[IBIS Ver]   5.0
[Comment Char] |_char
[File name]   dlpc231_ibis.ibs
[File Rev]   1.0
[Date]   August 11,2022
[Source]   Cadence SpeedXP Suite XtractIM 18.0.4.05011.160686   004
[Notes]   One-Section RLC
[Disclaimer]   The model given below represents a 201-pin package.
[Copyright]
[Component] Component_Name
[Manufacturer] Manufacturer_Name
[Package]
|   typ   min   max
R_pkg   0.29997   0.18892   0.43741
L_pkg   4.092e-9   2.338e-9   5.75e-9
C_pkg   1.277e-12   1.026e-12   1.843e-12
[Package Model]   dlpc231_pkg
[Pin]   Signal_name   model_name   R_pin   L_pin   C_pin
A1	GND18A_LVDS	GND
A10	DMD_LS0_CLK_N	fxslvtx-tx_n
A11	DMD_HS0_WDATA7_N	fxslvtx-tx_n
A12	DMD_HS0_WDATA6_N	fxslvtx-tx_n
A13	DMD_HS0_WDATA5_N	fxslvtx-tx_n
A14	DMD_HS0_WDATA4_N	fxslvtx-tx_n
A15	DMD_HS0_CLK_N	fxslvtx-tx_n
A16	DMD_HS0_WDATA3_N	fxslvtx-tx_n
A17	DMD_HS0_WDATA2_N	fxslvtx-tx_n
A18	GND18A_LVDS	GND
A2	DMD_HS1_WDATA2_N	fxslvtx-tx_n
A3	DMD_HS1_WDATA3_N	fxslvtx-tx_n
A4	DMD_HS1_CLK_N	fxslvtx-tx_n
A5	DMD_HS1_WDATA4_N	fxslvtx-tx_n
A6	DMD_HS1_WDATA5_N	fxslvtx-tx_n
A7	DMD_HS1_WDATA6_N	fxslvtx-tx_n
A8	DMD_HS1_WDATA7_N	fxslvtx-tx_n
A9	DMD_LS0_WDATA_N	fxslvtx-tx_n
B1	VCC18A_LVDS	POWER
B10	DMD_LS0_CLK_P	fxslvtx-tx_p
B11	DMD_HS0_WDATA7_P	fxslvtx-tx_p
B12	DMD_HS0_WDATA6_P	fxslvtx-tx_p
B13	DMD_HS0_WDATA5_P	fxslvtx-tx_p
B14	DMD_HS0_WDATA4_P	fxslvtx-tx_p
B15	DMD_HS0_CLK_P	fxslvtx-tx_p
B16	DMD_HS0_WDATA3_P	fxslvtx-tx_p
B17	DMD_HS0_WDATA2_P	fxslvtx-tx_p
B18	VCC18A_LVDS	POWER
B2	DMD_HS1_WDATA2_P	fxslvtx-tx_p
B3	DMD_HS1_WDATA3_P	fxslvtx-tx_p
B4	DMD_HS1_CLK_P	fxslvtx-tx_p
B5	DMD_HS1_WDATA4_P	fxslvtx-tx_p
B6	DMD_HS1_WDATA5_P	fxslvtx-tx_p
B7	DMD_HS1_WDATA6_P	fxslvtx-tx_p
B8	DMD_HS1_WDATA7_P	fxslvtx-tx_p
B9	DMD_LS0_WDATA_P	fxslvtx-tx_p
C1	DMD_HS1_WDATA1_N	fxslvtx-tx_n
C10	VCC11AD_PLLD	POWER
C11	GND11AD_PLLM	GND
C12	GNDIOLA_COSC	GND
C13	OSC_BYPASS	xtrnla
C14	GND18A_LVDS	GND
C15	VCC18A_LVDS	POWER
C16	GND18A_LVDS	GND
C17	DMD_HS0_WDATA1_P	fxslvtx-tx_p
C18	DMD_HS0_WDATA1_N	fxslvtx-tx_n
C2	DMD_HS1_WDATA1_P	fxslvtx-tx_p
C3	GND18A_LVDS	GND
C4	VCC18A_LVDS	POWER
C5	GND18A_LVDS	GND
C6	VCC18A_LVDS	POWER
C7	DMD_LS0_RDATA	xtrnla18
C8	DMD_LS1_RDATA	xtrnla18
C9	DMD_LS0_CLK	ztrfne4gsla18x1
D1	DMD_HS1_WDATA0_N	fxslvtx-tx_n
D10	GND11AD_PLLD	GND
D11	VCC11AD_PLLM	POWER
D12	PLL_REFCLK_I	NC
D13	PLL_REFCLK_O	NC
D14	VCC18A_LVDS	POWER
D15	RPI_0	NC
D16	VCC18A_LVDS	POWER
D17	DMD_HS0_WDATA0_P	fxslvtx-tx_p
D18	DMD_HS0_WDATA0_N	fxslvtx-tx_n
D2	DMD_HS1_WDATA0_P	fxslvtx-tx_p
D3	VCC18A_LVDS	POWER
D4	RPI_1	NC
D5	VCC18A_LVDS	POWER
D6	GND18A_LVDS	GND
D7	RPI_LS	NC
D8	DMD_LS0_WDATA	ztrfne4gsla18x1
D9	DMD_DEN_ARSTZ	ytrd4gsla18
E1	PMIC_LEDSEL_1	ztrnd28sla
E10	GND18A_LVDS	GND
E11	VCC3IO_COSC	POWER
E12	GND18A_LVDS	GND
E13	VCC18A_LVDS	POWER
E14	GND18A_LVDS	GND
E15	GPIO_31	ztrnd28sla
E16	GPIO_30	ztrnd28sla
E17	GPIO_29	ztrnd28sla
E18	GPIO_28	ztrnd28sla
E2	PMIC_INTZ	xtrnla
E3	PMIC_SPI_DIN	xtrnla
E4	PMIC_PARKZ	xtrnla
E5	PMIC_SPI_DOUT	ztrnd28sla
E6	VCC11A_DDI_1	POWER
E7	VCC11A_DDI_1	POWER
E8	GND18A_LVDS	GND
E9	VCC18IO	POWER
F1	PMIC_LEDSEL_3	ztrnd28sla
F10	VCC18A_LVDS	POWER
F11	VCCK	POWER
F12	VCC18A_LVDS	POWER
F13	VCC11A_DDI_0	POWER
F14	VCC3IO-2	POWER
F15	GPIO_27	ztrnd28sla
F16	GPIO_26	ztrnd28sla
F17	JTAGTDO3	ztrnd28sla
F18	JTAGTDO2	ztrnd28sla
F2	PMIC_LEDSEL_2	ztrnd28sla
F3	RESETZ	xtrnela
F4	PMIC_LEDSEL_0	ztrnd28sla
F5	PMIC_SPI_CLK	ztrnd28sla
F6	GND18A_LVDS	GND
F7	VCC18A_LVDS	POWER
F8	VCC18A_LVDS	POWER
F9	VCCK	POWER
G1	PMIC_AD3_CLK	ytrd28sla
G10	GND	GND
G11	GND	GND
G12	GND	GND
G13	VCC11A_DDI_0	POWER
G14	VCC3IO-2	POWER
G15	JTAGTDO1	ztrnd28sla
G16	JTAGTRSTZ	xtrnela
G17	JTAGTDI	xtrnla
G18	JTAGTMS3	xtrnla
G2	PMIC_AD3_MISO	xtrnla
G3	PMIC_AD3_MOSI	ztrnd28sla
G4	PMIC_SPI_CSZ_0	ztrnd28sla
G5	VCC3IO_MVGP	POWER
G6	VCCK	POWER
G7	GND	GND
G8	GND	GND
G9	GND	GND
H1	GPIO_02	ztrnd28sla
H10	GND	GND
H11	GND	GND
H12	GND	GND
H13	VCCK	POWER
H14	VCC3IO_INTF	POWER
H15	JTAGTMS2	xtrnla
H16	JTAGTMS1	xtrnla
H17	JTAGTCK	xtrnla
H18	HSYNC	ztrnd4gsla
H2	GPIO_05	ztrnd28sla
H3	GPIO_04	ztrnd28sla
H4	GPIO_00	ztrnd28sla
H5	VCC3IO_MVGP	POWER
H6	GND	GND
H7	GND	GND
H8	GND	GND
H9	GND	GND
J1	GPIO_01	ztrnd28sla
J10	GND	GND
J11	GND	GND
J12	GND	GND
J13	GND	GND
J14	VCC3IO_INTF	POWER
J15	PDATA_23	ztrnd4gsla
J16	PDATA_22	ztrnd4gsla
J17	PDATA_21	ztrnd4gsla
J18	VSYNC	ztrnd4gsla
J2	GPIO_03	ztrnd28sla
J3	GPIO_06	ztrnd28sla
J4	GPIO_07	ztrnd28sla
J5	HWTEST_EN	xtrnla
J6	VCCK	POWER
J7	GND	GND
J8	GND	GND
J9	GND	GND
K1	GPIO_08	ztrnd28sla
K10	GND	GND
K11	GND	GND
K12	GND	GND
K13	VCCK	POWER
K14	GND	GND
K15	PDATA_20	ztrnd4gsla
K16	PDATA_19	ztrnd4gsla
K17	PDATA_18	ztrnd4gsla
K18	PDATA_17	ztrnd4gsla
K2	GPIO_09	ztrnd28sla
K3	GPIO_10	ztrnd28sla
K4	GPIO_11	ztrnd28sla
K5	GPIO_12	ztrnd28sla
K6	VCC3IO	POWER
K7	GND	GND
K8	GND	GND
K9	GND	GND
L1	GPIO_13	ztrnd28sla
L10	GND	GND
L11	GND	GND
L12	GND	GND
L13	GND	GND
L14	VCC3IO_INTF	POWER
L15	HOST_IIC_SDA	ztriicla
L16	PDATA_16	ztrnd4gsla
L17	PDATA_15	ztrnd4gsla
L18	PDATA_14	ztrnd4gsla
L2	GPIO_14	ztrnd28sla
L3	GPIO_15	ztrnd28sla
L4	GPIO_16	ztrnd28sla
L5	VCC3IO	POWER
L6	VCCK	POWER
L7	GND	GND
L8	GND	GND
L9	GND	GND
M1	GPIO_17	ztrnd28sla
M10	GND	GND
M11	GND	GND
M12	GND	GND
M13	VCCK	POWER
M14	VCC3IO_INTF	POWER
M15	HOST_IIC_SCL	ztriicla
M16	PDATA_13	ztrnd4gsla
M17	DATEN	ztrnd4gsla
M18	PCLK	ztrnd4gsla
M2	GPIO_18	ztrnd28sla
M3	GPIO_19	ztrnd28sla
M4	GPIO_20	ztrnd28sla
M5	GPIO_24	ztrnd28sla
M6	VCC3IO	POWER
M7	GND	GND
M8	GND	GND
M9	GND	GND
N1	HOST_IF_SEL	ztrnd28sla
N10	VCC11A_LVDS	POWER
N11	VCCK	POWER
N12	GND	GND
N13	GND	GND
N14	GND	GND
N15	HOST_IRQ	ytrd28sla
N16	PDATA_11	ztrnd4gsla
N17	PDATA_12	ztrnd4gsla
N18	PDATA_9	ztrnd4gsla
N2	GPIO_21	ztrnd28sla
N3	GPIO_22	ztrnd28sla
N4	GPIO_23	ztrnd28sla
N5	VCC3IO_FLSH	POWER
N6	VCCK	POWER
N7	VCC3IO	POWER
N8	VCCK	POWER
N9	VCCK	POWER
P1	FLSH_SPI_DIO_0	ztrnd28sla
P10	EFUSE_POR33	NC
P11	VCC11A_LVDS	POWER
P12	VCC11A_LVDS	POWER
P13	VCC11A_LVDS	POWER
P14	VCC11A_LVDS	POWER
P15	HOST_SPI_DOUT	ytrd28sla
P16	PDATA_10	ztrnd4gsla
P17	PDATA_7	ztrnd4gsla
P18	PDATA_8	ztrnd4gsla
P2	HOST_SPI_MODE	ztrnd28sla
P3	GPIO_25	ztrnd28sla
P4	TSTPT_4	ztrnd4gsla
P5	VCC3IO_FLSH	POWER
P6	TSTPT_6	ztrnd4gsla
P7	TSTPT_7	ztrnd4gsla
P8	VCC3IO	POWER
P9	EFUSE_VDDQ	POWER
R1	FLSH_SPI_DIO_2	ztrnd28sla
R10	ETM_TRACECLK	ztrnd4gsla
R11	VCC33A_LVDS	POWER
R12	GND33A_LVDS	GND
R13	VCC33A_LVDS	POWER
R14	GND33A_LVDS	GND
R15	VCC33A_LVDS	POWER
R16	HOST_SPI_DIN	xtrnla
R17	PDATA_5	ztrnd4gsla
R18	PDATA_6	ztrnd4gsla
R2	FLSH_SPI_DIO_1	ztrnd28sla
R3	TSTPT_0	ztrnd4gsla
R4	TSTPT_1	ztrnd4gsla
R5	TSTPT_2	ztrnd4gsla
R6	MSTR_SCL	ztriicla
R7	TSTPT_3	ztrnd4gsla
R8	TSTPT_5	ztrnd4gsla
R9	ETM_TRACECTL	ztrnd4gsla
T1	FLSH_SPI_CSZ	ytrd28sla
T10	VCC33A_LVDS	POWER
T11	GND33A_LVDS	GND
T12	VCC33A_LVDS	POWER
T13	GND33A_LVDS	GND
T14	VCC33A_LVDS	POWER
T15	GND33A_LVDS	GND
T16	HOST_SPI_CSZ	xtrnla
T17	PDATA_3	ztrnd4gsla
T18	PDATA_4	ztrnd4gsla
T2	FLSH_SPI_DIO_3	ztrnd28sla
T3	VCC33A_LVDS	POWER
T4	VCC33A_LVDS	POWER
T5	GND33A_LVDS	GND
T6	GND33A_LVDS	GND
T7	MSTR_SDA	ztriicla
T8	VCC33A_LVDS	POWER
T9	GND33A_LVDS	GND
U1	FLSH_SPI_CLK	ytrd28sla
U10	L2_DATA0_N	fxlvrx-rx_n
U11	L2_DATA1_N	fxlvrx-rx_n
U12	L2_CLK_N	fxlvrx-rx_n
U13	L2_DATA2_N	fxlvrx-rx_n
U14	L2_DATA3_N	fxlvrx-rx_n
U15	GND33A_LVDS	GND
U16	HOST_SPI_CLK	xtrnla
U17	PDATA_1	ztrnd4gsla
U18	PDATA_2	ztrnd4gsla
U2	RTPPUB_ENZ	ztrnd28sla
U3	GND33A_LVDS	GND
U4	L1_DATA0_N	fxlvrx-rx_n
U5	L1_DATA1_N	fxlvrx-rx_n
U6	L1_CLK_N	fxlvrx-rx_n
U7	L1_DATA2_N	fxlvrx-rx_n
U8	L1_DATA3_N	fxlvrx-rx_n
U9	GND33A_LVDS	GND
V1	GND	GND
V10	L2_DATA0_P	fxlvrx-rx_p
V11	L2_DATA1_P	fxlvrx-rx_p
V12	L2_CLK_P	fxlvrx-rx_p
V13	L2_DATA2_P	fxlvrx-rx_p
V14	L2_DATA3_P	fxlvrx-rx_p
V15	GND33A_LVDS	GND
V16	VCC33A_LVDS	POWER
V17	PDATA_0	ztrnd4gsla
V18	GND	GND
V2	CRCZ_CHKSM_SEL	ztrnd28sla
V3	GND33A_LVDS	GND
V4	L1_DATA0_P	fxlvrx-rx_p
V5	L1_DATA1_P	fxlvrx-rx_p
V6	L1_CLK_P	fxlvrx-rx_p
V7	L1_DATA2_P	fxlvrx-rx_p
V8	L1_DATA3_P	fxlvrx-rx_p
V9	GND33A_LVDS	GND
| End of [PIN]
| ODT=0 DLPC230 internal termination is not enabled
| ODT=1 DLPC230 internal termination is enabled
|[Model Selector] fxlvrx-rx_p
|fxlvrx020hh0l-odt1-rx_p  ODT=1 mode
|fxlvrx020hh0l-odt0-rx_p  ODT=0 mode
|[Model Selector] fxlvrx-rx_n
|fxlvrx020hh0l-odt1-rx_n  ODT=1 mode
|fxlvrx020hh0l-odt0-rx_n  ODT=0 mode
[model selector]   ztrfne4gsla18x1
ztrfne4gsla18x1_1p8f 1.8mA bi-dir buffer
ztrfne4gsla18x1_1p8s 1.8mA bi-dir buffer
ztrfne4gsla18x1_3p6f 3.6mA bi-dir buffer
ztrfne4gsla18x1_3p6s 3.6mA bi-dir buffer
ztrfne4gsla18x1_5p4f 5.4mA bi-dir buffer
ztrfne4gsla18x1_5p4s 5.4mA bi-dir buffer
ztrfne4gsla18x1_7p2f 7.2mA bi-dir buffer
ztrfne4gsla18x1_7p2s 7.2mA bi-dir buffer
[model selector]   ztrnd4gsla
ztrnd4gsla_8f   8mA   bi-dir buffer   fast slew
ztrnd4gsla_12f   12mA  bi-dir buffer   fast slew
ztrnd4gsla_12s   12mA  bi-dir buffer   slow slew
ztrnd4gsla_16f   16mA  bi-dir buffer   fast slew
ztrnd4gsla_16s   16mA  bi-dir buffer   slow slew
ztrnd4gsla_4f   4mA   bi-dir buffer   fast slew
ztrnd4gsla_4s   4mA   bi-dir buffer   slow slew
ztrnd4gsla_8s   8mA   bi-dir buffer   slow slew
[model selector]   ztrnd28sla
ztrnd28sla_4f   4mA   bi-dir buffer   fast slew
ztrnd28sla_4s   4mA   bi-dir buffer   slow slew
ztrnd28sla_6f   6mA   bi-dir buffer   fast slew
ztrnd28sla_6s   6mA   bi-dir buffer   slow slew
ztrnd28sla_8f   8mA   bi-dir buffer   fast slew
ztrnd28sla_8s   8mA   bi-dir buffer   slow slew
ztrnd28sla_2f   2mA   bi-dir buffer   fast slew
ztrnd28sla_2s   2mA   bi-dir buffer   slow slew
[model selector]   ytrd28sla
ytrd28sla_4f   4mA   output buffer   fast slew
ytrd28sla_4s   4mA   output buffer   slow slew
ytrd28sla_6f   6mA   output buffer   fast slew
ytrd28sla_6s   6mA   output buffer   slow slew
ytrd28sla_8f   8mA   output buffer   fast slew
ytrd28sla_8s   8mA   output buffer   slow slew
ytrd28sla_2f   2mA   output buffer   fast slew
ytrd28sla_2s   2mA   output buffer   slow slew
[model selector]   ytrd4gsla18
ytrd4gsla18_1p5f   1.5mA output buffer   fast slew
ytrd4gsla18_1p5s   1.5mA output buffer   slow slew
ytrd4gsla18_3f   3mA   output buffer   fast slew
ytrd4gsla18_3s   3mA   output buffer   slow slew
ytrd4gsla18_4p5f   4.5mA output buffer   fast slew
ytrd4gsla18_4p5s   4.5mA output buffer   slow slew
ytrd4gsla18_6f   6mA   output buffer   fast slew
ytrd4gsla18_6s   6mA   output buffer   slow slew
[Define Package Model]   dlpc231_pkg
[Manufacturer]   TI
[OEM]   TI
[Description]   201-pin Package
|[Number of Sections]   1
[Number of Pins]   201
[Pin Numbers]
|[Pin Name]  Net Number   Net Name   Net's All Pins
P9   | 1   EFUSE_VDDQ   P9
K6   | 2   VCC3IO   K6
   |L5
   |M6
   |N7
   |P8
F14   | 3   VCC3IO-2   F14
   |G14
E11   | 4   VCC3IO_COSC   E11
N5   | 5   VCC3IO_FLSH   N5
   |P5
H14   | 6   VCC3IO_INTF   H14
   |J14
   |L14
   |M14
G5   | 7   VCC3IO_MVGP   G5
   |H5
C10   | 8   VCC11AD_PLLD   C10
D11   | 9   VCC11AD_PLLM   D11
F13   | 10   VCC11A_DDI_0   F13
   |G13
E6   | 11   VCC11A_DDI_1   E6
   |E7
N10   | 12   VCC11A_LVDS   N10
   |P11
   |P12
   |P13
   |P14
B1   | 13   VCC18A_LVDS   B1
   |B18
   |C4
   |C6
   |C15
   |D3
   |D5
   |D14
   |D16
   |E13
   |F7
   |F8
   |F10
   |F12
E9   | 14   VCC18IO   E9
R11   | 15   VCC33A_LVDS   R11
   |R13
   |R15
   |T3
   |T4
   |T8
   |T10
   |T12
   |T14
   |V16
F9   | 16   VCCK   F9
   |F11
   |G6
   |H13
   |J6
   |K13
   |L6
   |M13
   |N6
   |N8
   |N9
   |N11
V2   | 17   CRCZ_CHKSM_SEL   V2
M17   | 18   DATEN   M17
D9   | 19   DMD_DEN_ARSTZ   D9
A15   | 20   DMD_HS0_CLK_N   A15
B15   | 21   DMD_HS0_CLK_P   B15
D18   | 22   DMD_HS0_WDATA0_N   D18
D17   | 23   DMD_HS0_WDATA0_P   D17
C18   | 24   DMD_HS0_WDATA1_N   C18
C17   | 25   DMD_HS0_WDATA1_P   C17
A17   | 26   DMD_HS0_WDATA2_N   A17
B17   | 27   DMD_HS0_WDATA2_P   B17
A16   | 28   DMD_HS0_WDATA3_N   A16
B16   | 29   DMD_HS0_WDATA3_P   B16
A14   | 30   DMD_HS0_WDATA4_N   A14
B14   | 31   DMD_HS0_WDATA4_P   B14
A13   | 32   DMD_HS0_WDATA5_N   A13
B13   | 33   DMD_HS0_WDATA5_P   B13
A12   | 34   DMD_HS0_WDATA6_N   A12
B12   | 35   DMD_HS0_WDATA6_P   B12
A11   | 36   DMD_HS0_WDATA7_N   A11
B11   | 37   DMD_HS0_WDATA7_P   B11
A4   | 38   DMD_HS1_CLK_N   A4
B4   | 39   DMD_HS1_CLK_P   B4
D1   | 40   DMD_HS1_WDATA0_N   D1
D2   | 41   DMD_HS1_WDATA0_P   D2
C1   | 42   DMD_HS1_WDATA1_N   C1
C2   | 43   DMD_HS1_WDATA1_P   C2
A2   | 44   DMD_HS1_WDATA2_N   A2
B2   | 45   DMD_HS1_WDATA2_P   B2
A3   | 46   DMD_HS1_WDATA3_N   A3
B3   | 47   DMD_HS1_WDATA3_P   B3
A5   | 48   DMD_HS1_WDATA4_N   A5
B5   | 49   DMD_HS1_WDATA4_P   B5
A6   | 50   DMD_HS1_WDATA5_N   A6
B6   | 51   DMD_HS1_WDATA5_P   B6
A7   | 52   DMD_HS1_WDATA6_N   A7
B7   | 53   DMD_HS1_WDATA6_P   B7
A8   | 54   DMD_HS1_WDATA7_N   A8
B8   | 55   DMD_HS1_WDATA7_P   B8
C9   | 56   DMD_LS0_CLK   C9
A10   | 57   DMD_LS0_CLK_N   A10
B10   | 58   DMD_LS0_CLK_P   B10
C7   | 59   DMD_LS0_RDATA   C7
D8   | 60   DMD_LS0_WDATA   D8
A9   | 61   DMD_LS0_WDATA_N   A9
B9   | 62   DMD_LS0_WDATA_P   B9
C8   | 63   DMD_LS1_RDATA   C8
P10   | 64   EFUSE_POR33   P10
R10   | 65   ETM_TRACECLK   R10
R9   | 66   ETM_TRACECTL   R9
U1   | 67   FLSH_SPI_CLK   U1
T1   | 68   FLSH_SPI_CSZ   T1
P1   | 69   FLSH_SPI_DIO_0   P1
R2   | 70   FLSH_SPI_DIO_1   R2
R1   | 71   FLSH_SPI_DIO_2   R1
T2   | 72   FLSH_SPI_DIO_3   T2
H4   | 73   GPIO_00   H4
J1   | 74   GPIO_01   J1
H1   | 75   GPIO_02   H1
J2   | 76   GPIO_03   J2
H3   | 77   GPIO_04   H3
H2   | 78   GPIO_05   H2
J3   | 79   GPIO_06   J3
J4   | 80   GPIO_07   J4
K1   | 81   GPIO_08   K1
K2   | 82   GPIO_09   K2
K3   | 83   GPIO_10   K3
K4   | 84   GPIO_11   K4
K5   | 85   GPIO_12   K5
L1   | 86   GPIO_13   L1
L2   | 87   GPIO_14   L2
L3   | 88   GPIO_15   L3
L4   | 89   GPIO_16   L4
M1   | 90   GPIO_17   M1
M2   | 91   GPIO_18   M2
M3   | 92   GPIO_19   M3
M4   | 93   GPIO_20   M4
N2   | 94   GPIO_21   N2
N3   | 95   GPIO_22   N3
N4   | 96   GPIO_23   N4
M5   | 97   GPIO_24   M5
P3   | 98   GPIO_25   P3
F16   | 99   GPIO_26   F16
F15   | 100   GPIO_27   F15
E18   | 101   GPIO_28   E18
E17   | 102   GPIO_29   E17
E16   | 103   GPIO_30   E16
E15   | 104   GPIO_31   E15
N1   | 105   HOST_IF_SEL   N1
M15   | 106   HOST_IIC_SCL   M15
L15   | 107   HOST_IIC_SDA   L15
N15   | 108   HOST_IRQ   N15
U16   | 109   HOST_SPI_CLK   U16
T16   | 110   HOST_SPI_CSZ   T16
R16   | 111   HOST_SPI_DIN   R16
P15   | 112   HOST_SPI_DOUT   P15
P2   | 113   HOST_SPI_MODE   P2
H18   | 114   HSYNC   H18
J5   | 115   HWTEST_EN   J5
H17   | 116   JTAGTCK   H17
G17   | 117   JTAGTDI   G17
G15   | 118   JTAGTDO1   G15
F18   | 119   JTAGTDO2   F18
F17   | 120   JTAGTDO3   F17
H16   | 121   JTAGTMS1   H16
H15   | 122   JTAGTMS2   H15
G18   | 123   JTAGTMS3   G18
G16   | 124   JTAGTRSTZ   G16
U6   | 125   L1_CLK_N   U6
V6   | 126   L1_CLK_P   V6
U4   | 127   L1_DATA0_N   U4
V4   | 128   L1_DATA0_P   V4
U5   | 129   L1_DATA1_N   U5
V5   | 130   L1_DATA1_P   V5
U7   | 131   L1_DATA2_N   U7
V7   | 132   L1_DATA2_P   V7
U8   | 133   L1_DATA3_N   U8
V8   | 134   L1_DATA3_P   V8
U12   | 135   L2_CLK_N   U12
V12   | 136   L2_CLK_P   V12
U10   | 137   L2_DATA0_N   U10
V10   | 138   L2_DATA0_P   V10
U11   | 139   L2_DATA1_N   U11
V11   | 140   L2_DATA1_P   V11
U13   | 141   L2_DATA2_N   U13
V13   | 142   L2_DATA2_P   V13
U14   | 143   L2_DATA3_N   U14
V14   | 144   L2_DATA3_P   V14
R6   | 145   MSTR_SCL   R6
T7   | 146   MSTR_SDA   T7
C13   | 147   OSC_BYPASS   C13
M18   | 148   PCLK   M18
V17   | 149   PDATA_0   V17
U17   | 150   PDATA_1   U17
U18   | 151   PDATA_2   U18
T17   | 152   PDATA_3   T17
T18   | 153   PDATA_4   T18
R17   | 154   PDATA_5   R17
R18   | 155   PDATA_6   R18
P17   | 156   PDATA_7   P17
P18   | 157   PDATA_8   P18
N18   | 158   PDATA_9   N18
P16   | 159   PDATA_10   P16
N16   | 160   PDATA_11   N16
N17   | 161   PDATA_12   N17
M16   | 162   PDATA_13   M16
L18   | 163   PDATA_14   L18
L17   | 164   PDATA_15   L17
L16   | 165   PDATA_16   L16
K18   | 166   PDATA_17   K18
K17   | 167   PDATA_18   K17
K16   | 168   PDATA_19   K16
K15   | 169   PDATA_20   K15
J17   | 170   PDATA_21   J17
J16   | 171   PDATA_22   J16
J15   | 172   PDATA_23   J15
D12   | 173   PLL_REFCLK_I   D12
D13   | 174   PLL_REFCLK_O   D13
G1   | 175   PMIC_AD3_CLK   G1
G2   | 176   PMIC_AD3_MISO   G2
G3   | 177   PMIC_AD3_MOSI   G3
E2   | 178   PMIC_INTZ   E2
F4   | 179   PMIC_LEDSEL_0   F4
E1   | 180   PMIC_LEDSEL_1   E1
F2   | 181   PMIC_LEDSEL_2   F2
F1   | 182   PMIC_LEDSEL_3   F1
E4   | 183   PMIC_PARKZ   E4
F5   | 184   PMIC_SPI_CLK   F5
G4   | 185   PMIC_SPI_CSZ_0   G4
E3   | 186   PMIC_SPI_DIN   E3
E5   | 187   PMIC_SPI_DOUT   E5
F3   | 188   RESETZ   F3
D15   | 189   RPI_0   D15
D4   | 190   RPI_1   D4
D7   | 191   RPI_LS   D7
U2   | 192   RTPPUB_ENZ   U2
R3   | 193   TSTPT_0   R3
R4   | 194   TSTPT_1   R4
R5   | 195   TSTPT_2   R5
R7   | 196   TSTPT_3   R7
P4   | 197   TSTPT_4   P4
R8   | 198   TSTPT_5   R8
P6   | 199   TSTPT_6   P6
P7   | 200   TSTPT_7   P7
J18   | 201   VSYNC   J18
[Model Data]
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[End Model Data]
[End Package Model]
| Models and submodels in the file (48): fxlvrx020hh0l-odt0-rx_p (Input), fxlvrx020hh0l-odt0-rx_n (Input), fxslvtx-tx_p (Output), fxslvtx-tx_n (Output), ztrfne4gsla18x1_1p8f (I/O), ztrfne4gsla18x1_1p8s (I/O), ztrfne4gsla18x1_3p6f (I/O), ztrfne4gsla18x1_3p6s (I/O), ztrfne4gsla18x1_5p4f (I/O), ztrfne4gsla18x1_5p4s (I/O), ztrfne4gsla18x1_7p2f (I/O), ztrfne4gsla18x1_7p2s (I/O), ztrnd4gsla_8f (I/O), ztrnd4gsla_12f (I/O), ztrnd4gsla_12s (I/O), ztrnd4gsla_16f (I/O), ztrnd4gsla_16s (I/O), ztrnd4gsla_4f (I/O), ztrnd4gsla_4s (I/O), ztrnd4gsla_8s (I/O), ztrnd28sla_4f (I/O), ztrnd28sla_4s (I/O), ztrnd28sla_6f (I/O), ztrnd28sla_6s (I/O), ztrnd28sla_8f (I/O), ztrnd28sla_8s (I/O), ztrnd28sla_2f (I/O), ztrnd28sla_2s (I/O), ytrd28sla_4f (3-state), ytrd28sla_4s (3-state), ytrd28sla_6f (3-state), ytrd28sla_6s (3-state), ytrd28sla_8f (3-state), ytrd28sla_8s (3-state), ytrd28sla_2f (3-state), ytrd28sla_2s (3-state), xtrnla (Input), xtrnla18 (Input), ytrd4gsla18_1p5f (3-state), ytrd4gsla18_1p5s (3-state), ytrd4gsla18_3f (3-state), ytrd4gsla18_3s (3-state), ytrd4gsla18_4p5f (3-state), ytrd4gsla18_4p5s (3-state), ytrd4gsla18_6f (3-state), ytrd4gsla18_6s (3-state), xtrnela (Input), ztriicla (I/O_open_drain)
